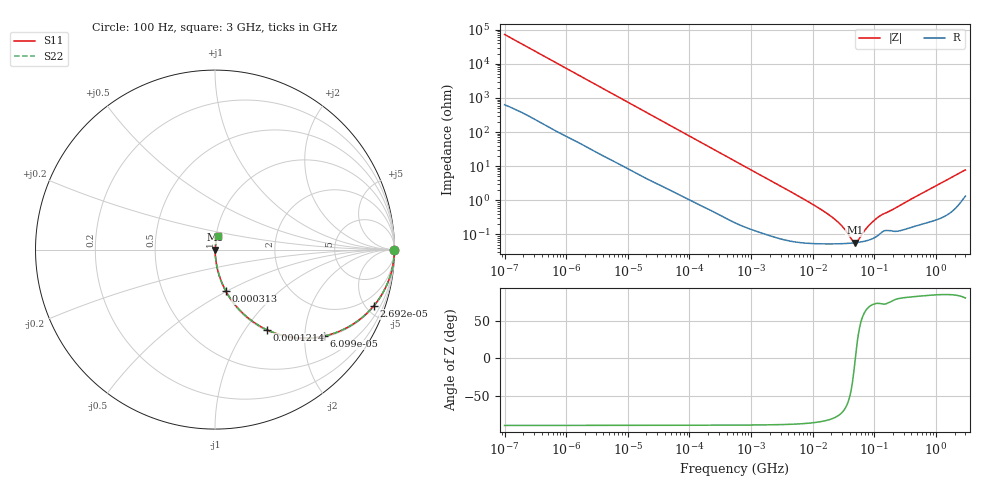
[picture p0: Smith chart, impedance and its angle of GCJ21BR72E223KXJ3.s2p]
!Murata Part Number: GCJ21BR72E223KXJ3
!These Parameters are Measured in Series Mode Connection
!Data Generated on Mar 13, 2026
!  o--ll--o
!Port1  Port2
!  o------o
!Operation Temp=25[degC], DC Bias Voltage=0[V]
!Freq. Start=100[Hz] Stop=3[GHz] 401[Steps]
# Hz S RI R 50
!Freq.(Hz) S11(Real) S11(Imag) S21(Real) S21(Imag) S12(Real) S12(Imag) S22(Real) S22(Imag)
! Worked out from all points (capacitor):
!   401 points, 100 Hz to 3 GHz, reference 50 ohm
!   read as one part in series: C = 21.8 nF near 109 Hz
!   lowest |Z| = 57.1 mohm at 48.15 MHz (marker M1)
!   series resonance near 49.16 MHz, so ESL is about 480 pH
!   S11 on the Smith chart (normalised r, x): 100 Hz: open; 26.92 kHz: 1.07, -5.63; 60.99 kHz: 1.03, -2.50; 121.4 kHz: 1.02, -1.26; 313 kHz: 1.01, -0.49; 3 GHz: 1.03, +0.15
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100  1 -0.00137  1.38e-05 0.00137  1.38e-05 0.00137  1 -0.00137
1788  0.9992 -0.024  0.000831 0.024  0.000831 0.024  0.9992 -0.024
8421  0.9864 -0.1104  0.0136 0.1104  0.0136 0.1104  0.9864 -0.1104
26919  0.8849 -0.3133  0.1151 0.3133  0.1151 0.3133  0.8849 -0.3133
31977  0.846 -0.355  0.154 0.355  0.154 0.355  0.846 -0.355
60986  0.6083 -0.4818  0.3917 0.4818  0.3917 0.4818  0.6083 -0.4818
121426  0.2874 -0.4459  0.7126 0.4459  0.7126 0.4459  0.2874 -0.4459
186741  0.1486 -0.3486  0.8514 0.3486  0.8514 0.3486  0.1486 -0.3486
313007  0.0605 -0.2311  0.9395 0.2311  0.9395 0.2311  0.0605 -0.2311
547723  0.0217 -0.1383  0.9783 0.1383  0.9783 0.1383  0.0217 -0.1383
1677156  0.00318 -0.0464  0.9968 0.0464  0.9968 0.0464  0.00318 -0.0464
9794414  0.000598 -0.00773  0.9994 0.00773  0.9994 0.00773  0.000598 -0.00773
2.52476e7  0.000534 -0.0023  0.9995 0.0023  0.9995 0.0023  0.000534 -0.0023
3.268714e7  0.000539 -0.00135  0.9995 0.00135  0.9995 0.00135  0.000539 -0.00135
4.418008e7  0.000558 -0.000343  0.9994 0.000343  0.9994 0.000343  0.000558 -0.000343
4.815176e7  0.000567 -6.59e-05  0.9994 6.59e-05  0.9994 6.59e-05  0.000567 -6.59e-05
5.478864e7  0.000584 0.000349  0.9994 -0.000349  0.9994 -0.000349  0.000584 0.000349
7.405258e7  0.000651 0.00135  0.9993 -0.00135  0.9993 -0.00135  0.000651 0.00135
9.587315e7  0.00077 0.00231  0.9992 -0.00231  0.9992 -0.00231  0.00077 0.00231
1.241234e8  0.00106 0.00336  0.9989 -0.00336  0.9989 -0.00336  0.00106 0.00336
1.751444e8  0.00131 0.00458  0.9987 -0.00458  0.9987 -0.00458  0.00131 0.00458
3e9  0.0186 0.0739  0.9814 -0.0739  0.9814 -0.0739  0.0186 0.0739
